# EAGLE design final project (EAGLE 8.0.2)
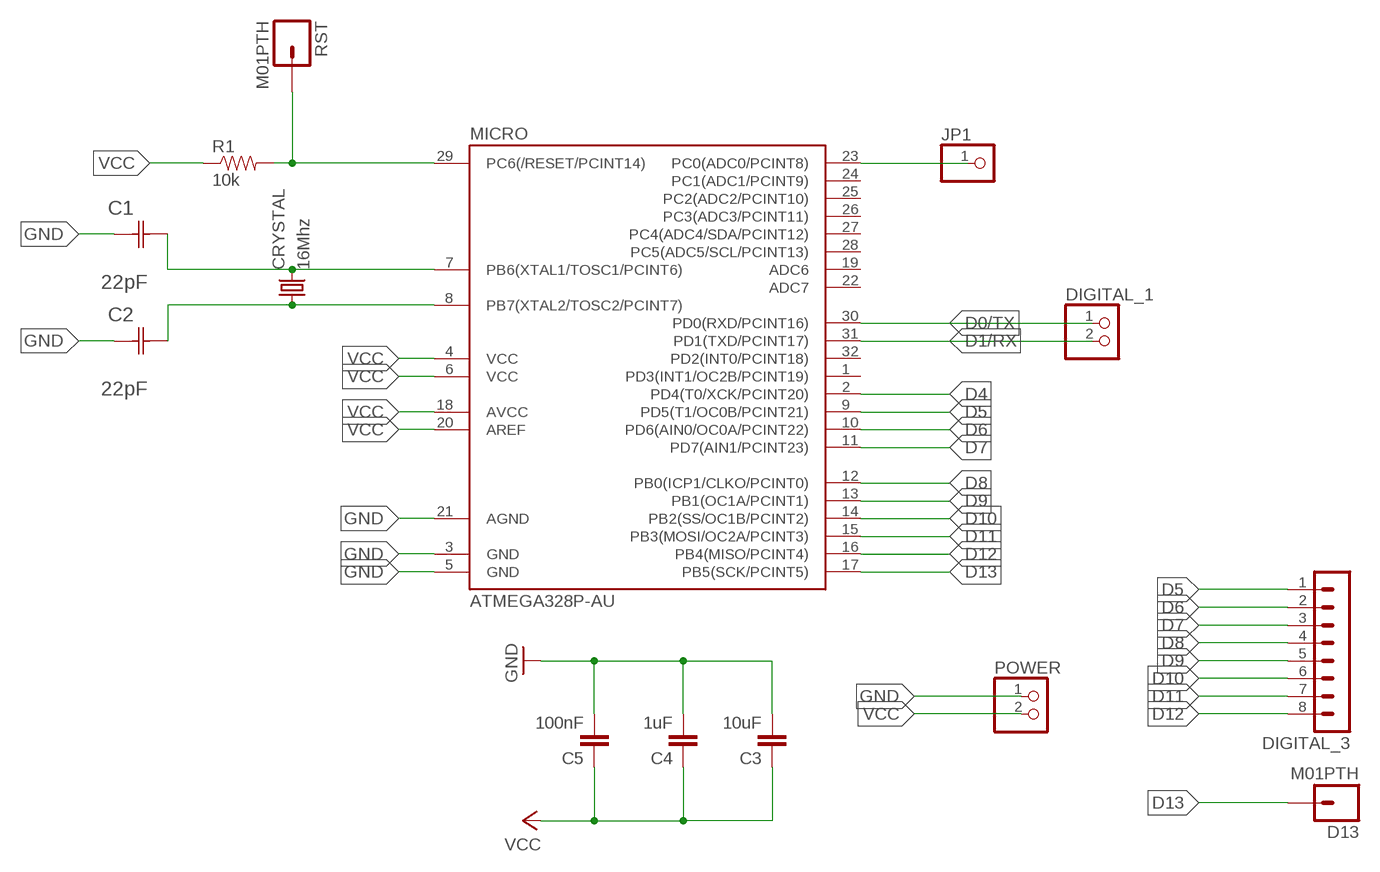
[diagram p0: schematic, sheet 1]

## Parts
C1  22pF  0612ZC225MAT2A  [CAPC3216X178N]
C2  22pF  0612ZC225MAT2A  [CAPC3216X178N]
C3  10uF  CAP1206  [1206]
C4  1uF  CAP1206  [1206]
C5  100nF  CAP1206  [1206]
CRYSTAL  16Mhz  CSM-7X-DU  [CSM-7X-DU]
D13  M01PTH  [1X01]
DIGITAL_1  PINHD-1X2  [1X02]
DIGITAL_3  MA08-1  [MA08-1]
JP1  PINHD-1X1  [1X01]
MICRO  ATMEGA328P-AU  ATMEGA48/88/168-AU  [TQFP32-08]
POWER  PINHD-1X2  [1X02]
R1  10k  RESISTOR1206  [1206]
RST  M01PTH  [1X01]

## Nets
D0/TX: DIGITAL_1.1 MICRO.30(PD0(RXD/PCINT16))
D1/RX: DIGITAL_1.2 MICRO.31(PD1(TXD/PCINT17))
D4: MICRO.2(PD4(T0/XCK/PCINT20))
D5: DIGITAL_3.1 MICRO.9(PD5(T1/OC0B/PCINT21))
D6: DIGITAL_3.2 MICRO.10(PD6(AIN0/OC0A/PCINT22))
D7: DIGITAL_3.3 MICRO.11(PD7(AIN1/PCINT23))
D8: DIGITAL_3.4 MICRO.12(PB0(ICP1/CLKO/PCINT0))
D9: DIGITAL_3.5 MICRO.13(PB1(OC1A/PCINT1))
D10: DIGITAL_3.6 MICRO.14(PB2(SS/OC1B/PCINT2))
D11: DIGITAL_3.7 MICRO.15(PB3(MOSI/OC2A/PCINT3))
D12: DIGITAL_3.8 MICRO.16(PB4(MISO/PCINT4))
D13: D13.1 MICRO.17(PB5(SCK/PCINT5))
GND: C1.1(C1) C2.1(C1) C3.2 C4.2 C5.2 MICRO.3(GND) MICRO.5(GND) MICRO.21(AGND) POWER.1
N$1: JP1.1 MICRO.23(PC0(ADC0/PCINT8))
N$2: C1.2(C2) CRYSTAL.2 MICRO.7(PB6(XTAL1/TOSC1/PCINT6))
N$3: MICRO.29(PC6(/RESET/PCINT14)) R1.2 RST.1
N$9: C2.2(C2) CRYSTAL.1 MICRO.8(PB7(XTAL2/TOSC2/PCINT7))
VCC: C3.1 C4.1 C5.1 MICRO.4(VCC) MICRO.6(VCC) MICRO.18(AVCC) MICRO.20(AREF) POWER.2 R1.1
Unconnected: MICRO.1(PD3(INT1/OC2B/PCINT19)) MICRO.19(ADC6) MICRO.22(ADC7) MICRO.24(PC1(ADC1/PCINT9)) MICRO.25(PC2(ADC2/PCINT10)) MICRO.26(PC3(ADC3/PCINT11)) MICRO.27(PC4(ADC4/SDA/PCINT12)) MICRO.28(PC5(ADC5/SCL/PCINT13)) MICRO.32(PD2(INT0/PCINT18))

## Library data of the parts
C1 C2 = AVX_By_element14_Batch_1:0612ZC225MAT2A: Capacitor 1206; MPN: 0612ZC225MAT2A; OC_FARNELL: -; OC_NEWARK: 12N3209; SUPPLIER: AVX; TOLERANCE: ±20%; VALUE: 2.2µF; VOLTAGERATING: 10V
C3-C5 = 01_SparkFun:CAP: Capacitor
CRYSTAL = 01_FAB_Hello:CSM-7X-DU: SMD CRYSTAL; OC_FARNELL: unknown; OC_NEWARK: unknown
D13 RST = 01_SparkFun:M01: Header 1
DIGITAL_1 POWER = pinhead:PINHD-1X2: PIN HEADER
DIGITAL_3 = con-lstb:MA08-1: PIN HEADER; OC_FARNELL: unknown; OC_NEWARK: unknown
JP1 = pinhead:PINHD-1X1: PIN HEADER
MICRO = atmega8:ATMEGA48/88/168
R1 = 01_SparkFun:RESISTOR: Resistor

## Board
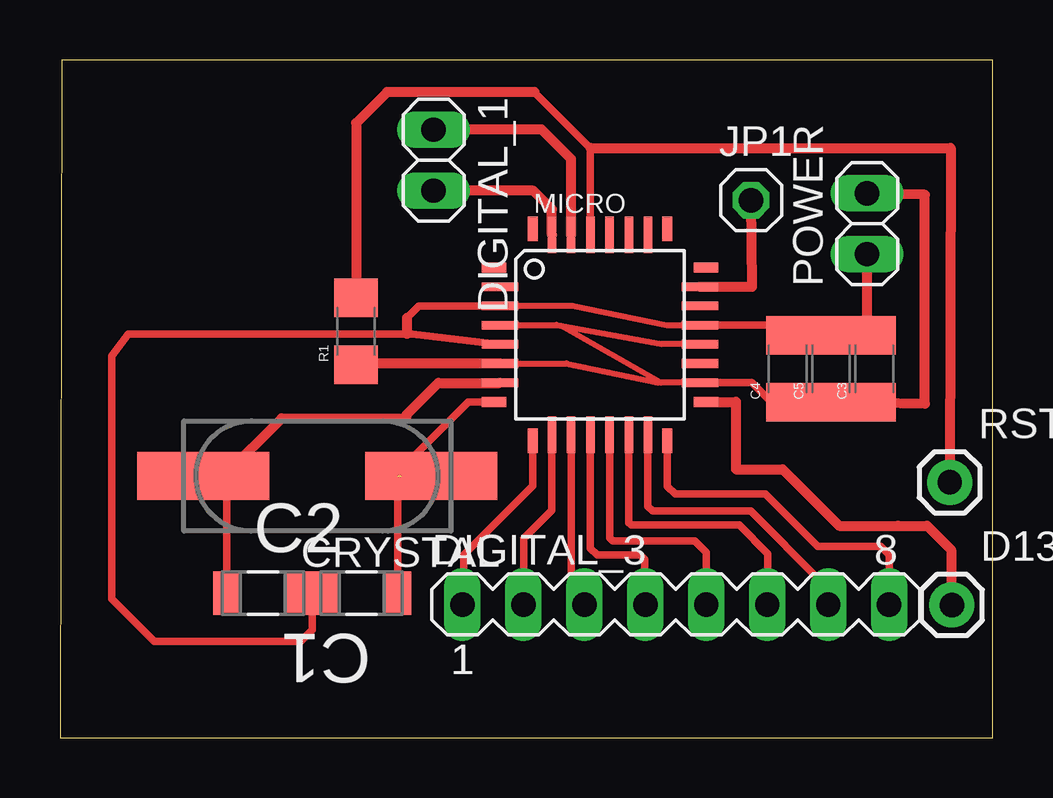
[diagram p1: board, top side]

Size 38.86 x 28.26 mm. Coordinates in mm from the lower left corner, seen from the top.
Outline: 0,0 38.86,0 38.86,28.26 0.08,28.26 0,0
Copper layers (1*16): Top 0.035mm / dielectric 1.5mm / Bottom 0.035mm
Design rules "default": minimum track width 10mil, minimum drill 24mil, track to track 8mil, track to pad 8mil, pad to pad 8mil, via to via 8mil, smd to smd 8mil, copper to edge 40mil, drill to drill 8mil, minimum pad ring 10mil, minimum via ring 8mil, stop-mask expansion 4mil, vias tented up to drill 0mil, thermal gap 10mil

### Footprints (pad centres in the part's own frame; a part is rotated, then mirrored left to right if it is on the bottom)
CAPC3216X178N = smd 1.118 x 1.803: 1 -1.499,0; 2 1.499,0
1206 = smd 1.6 x 1.8: 1 -1.4,0; 2 1.4,0
CSM-7X-DU = smd 5.5 x 2: 1 -4.75,0; 2 4.75,0
1X01 = drill 1.016 pad 1.88: 1 0,0
1X02 = drill 1.016 long: 1 -1.27,0; 2 1.27,0
MA08-1 = drill 1.016 long: 1 -8.89,0; 2 -6.35,0; 3 -3.81,0; 4 -1.27,0; 5 1.27,0; 6 3.81,0; 7 6.35,0; 8 8.89,0
1X01' = drill 1.016 octagon: 1 0,0
TQFP32-08 = smd 1.016 x 0.406: 1 -4.42,2.8; 8 -4.42,-2.8; 17 4.42,-2.8; 24 4.42,2.8 | smd 1.524 x 0.356: 2 -4.166,2; 3 -4.166,1.2; 4 -4.166,0.4; 5 -4.166,-0.4; 6 -4.166,-1.2; 7 -4.166,-2; 18 4.166,-2; 19 4.166,-1.2; 20 4.166,-0.4; 21 4.166,0.4; 22 4.166,1.2; 23 4.166,2 | smd 0.406 x 1.016: 9 -2.8,-4.42; 16 2.8,-4.42; 25 2.8,4.42; 32 -2.8,4.42 | smd 0.356 x 1.524: 10 -2,-4.166; 11 -1.2,-4.166; 12 -0.4,-4.166; 13 0.4,-4.166; 14 1.2,-4.166; 15 2,-4.166; 26 2,4.166; 27 1.2,4.166; 28 0.4,4.166; 29 -0.4,4.166; 30 -1.2,4.166; 31 -2,4.166

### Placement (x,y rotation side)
C1  8.45,6.04 180 top
C2  12.57,6.04 0 top
C3  33.93,15.38 90 top
C4  30.32,15.38 90 top
C5  32.13,15.38 90 top
CRYSTAL  10.71,10.91 180 top
D13  37.16,5.53 0 top
DIGITAL_1  15.57,24.08 270 top
DIGITAL_3  25.66,5.56 0 top
JP1  [1X01']  28.79,22.41 0 top
MICRO  22.5,16.8 0 top
POWER  33.63,21.44 90 top
R1  12.34,16.94 90 top
RST  37.07,10.65 0 top

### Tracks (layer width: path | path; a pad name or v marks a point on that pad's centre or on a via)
D0/TX
  Top 0.406: MICRO.30 21.3,24.13 20.07,25.36 DIGITAL_1.1
D1/RX
  Top 0.406: MICRO.31 20.5,22.04 19.72,22.81 DIGITAL_1.2
D5
  Top 0.305: MICRO.9 19.7,10.5 16.81,7.62 16.81,5.6 DIGITAL_3.1
D6
  Top 0.305: MICRO.10 20.5,9.48 19.33,8.31 19.33,5.58 DIGITAL_3.2
D7
  Top 0.305: MICRO.11 21.3,6.11 DIGITAL_3.3
D8
  Top 0.305: MICRO.12 22.1,7.9 22.38,7.62 24.18,7.62 24.36,7.44 24.36,5.59 DIGITAL_3.4
D9
  Top 0.305: MICRO.13 22.9,8.34 23.04,8.2 26.44,8.2 26.92,7.72 DIGITAL_3.5
D10
  Top 0.305: MICRO.14 23.7,8.96 23.8,8.87 28.3,8.87 29.49,7.67 29.49,5.58 DIGITAL_3.6
D11
  Top 0.305: MICRO.15 24.5,9.64 24.69,9.45 28.78,9.45 31.73,6.5 31.73,5.84 DIGITAL_3.7
D12
  Top 0.305: MICRO.16 25.3,10.49 25.63,10.16 29.39,10.16 31.57,7.98 34.19,7.98 34.54,7.62 DIGITAL_3.8
D13
  Top 0.406: MICRO.17 28.17,14.01 28.17,11.2 30.11,11.2 32.47,8.84 34.91,8.84 36.13,8.84 37.13,7.84 37.13,5.57 D13.1
GND
  Top 0.254: MICRO.21 26.65,17.19 25.29,17.19 21.35,18.01 MICRO.3
  Top 0.305: MICRO.21 29.9,17.2 C4.2 C5.2 C3.2 | MICRO.5 14.68,16.84 14.45,16.84 2.84,16.84 2.16,15.93 2.16,5.79 3.94,4.01 10.03,4.01 10.52,4.5 10.52,5.99 | 10.52,5.99 10.49,6.02 9.95,6.02 C1.1 | 10.52,5.99 11.07,5.99 C2.1 | MICRO.3 14.96,18.01 14.45,17.5
  Top 0.406: C3.2 33.63,16.78 POWER.1 | 14.45,17.5 14.45,16.84
N$1
  Top 0.406: MICRO.23 28.84,18.8 JP1.1
N$2
  Top 0.254: 6.96,10.33 6.6,10.68 6.19,10.68 CRYSTAL.2
  Top 0.305: C1.2 6.96,10.33
  Top 0.406: CRYSTAL.2 6.83,10.91 9.24,13.32 14.43,13.32 14.43,13.46 15.76,14.79 18.32,14.79 MICRO.7
N$3
  Top 0.305: MICRO.29 22.1,24.59 19.76,26.92
  Top 0.406: 22.1,24.59 37.11,24.59 RST.1 | 19.76,26.92 13.63,26.92 12.34,25.63 R1.2 | R1.2
N$9  (1 unrouted)
  Top 0.305: MICRO.8 17.01,14.01 13.88,10.87 13.88,10.91 14.21,10.91 CRYSTAL.1 | C2.2 14.07,10.91
VCC
  Top 0.254: MICRO.20 26.05,16.41 26.05,16.42 25.09,16.42 20.86,17.18 | MICRO.4 20.68,17.21 20.86,17.18 | 19.02,15.61 21.1,15.61 24.91,14.81 24.91,14.8 MICRO.18 | 26.67,14.81 MICRO.18 25.04,14.81 20.86,17.18
  Top 0.305: MICRO.18 | MICRO.20 26.05,16.42 | 26.66,14.77 MICRO.18 | 19.02,15.61 MICRO.6 | C5.1 C4.1 30.36,13.95 30.94,13.95 30.91,13.97 29.66,13.97 28.82,14.81 26.67,14.81 MICRO.18 | 31.98,13.84 C5.1 | C5.1 C3.1
  Top 0.406: C3.1 36.04,13.93 36.04,22.64 POWER.2 | MICRO.6 12.4,15.61 R1.1

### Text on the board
200bmp: C:/Users/Usuario/Desktop/DROT1.bmp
